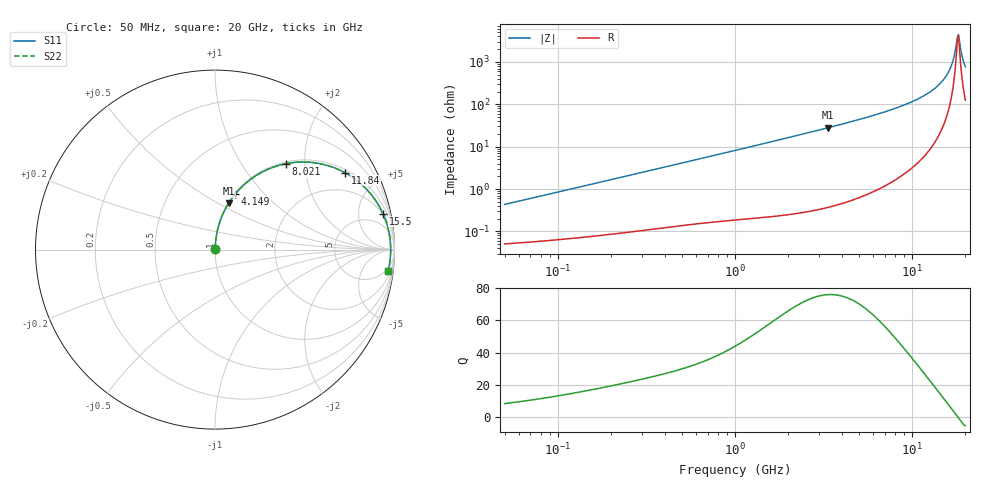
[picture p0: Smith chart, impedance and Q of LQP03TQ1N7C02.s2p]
!Murata Part Number: LQP03TQ1N7C02
!These Parameters are Measured in Series Mode Connection
!  o--[Z]--o
!Port1  Port2
!  o-------o
!Freq. Start=50[MHz] Stop=20[GHz], 401[Steps]
# Hz S RI R 50
!Freq.(Hz) S11(Real) S11(Imag) S21(Real) S21(Imag) S12(Real) S12(Imag) S22(Real) S22(Imag)
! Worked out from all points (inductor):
!   401 points, 50 MHz to 20 GHz, reference 50 ohm
!   read as one part in series: L = 1.36 nH near 51.52 MHz
!   highest Q = 75.9 at 3.364 GHz (marker M1), where L = 1.33 nH
!   self-resonance near 18.01 GHz
!   S11 on the Smith chart (normalised r, x): 50 MHz: 1.00, +0.01; 4.149 GHz: 1.01, +0.70; 8.021 GHz: 1.03, +1.60; 11.84 GHz: 1.12, +3.30; 15.5 GHz: 1.90, +9.01; 20 GHz: 4, -15
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5e7  0.000523 0.00429  0.9995 -0.00429  0.9995 -0.00429  0.000523 0.00429
1.364002e8  0.000849 0.0114  0.9992 -0.0114  0.9992 -0.0114  0.000849 0.0114
3.721004e8  0.0021 0.0305  0.9979 -0.0305  0.9979 -0.0305  0.0021 0.0305
1e9  0.00837 0.0804  0.9916 -0.0804  0.9916 -0.0804  0.00837 0.0804
2.728004e9  0.0507 0.2128  0.9493 -0.2128  0.9493 -0.2128  0.0507 0.2128
3.364474e9  0.0759 0.2583  0.9241 -0.2583  0.9241 -0.2583  0.0759 0.2583
4.149438e9  0.1137 0.3109  0.8863 -0.3109  0.8863 -0.3109  0.1137 0.3109
5.683258e9  0.208 0.3984  0.792 -0.3984  0.792 -0.3984  0.208 0.3984
7.442007e9  0.3438 0.4657  0.6562 -0.4657  0.6562 -0.4657  0.3438 0.4657
8.020766e9  0.3931 0.4784  0.6069 -0.4784  0.6069 -0.4784  0.3931 0.4784
9.892087e9  0.5592 0.4832  0.4408 -0.4832  0.4408 -0.4832  0.5592 0.4832
1.183995e10  0.7242 0.4284  0.2758 -0.4284  0.2758 -0.4284  0.7242 0.4284
1.375312e10  0.8554 0.3241  0.1446 -0.3241  0.1446 -0.3241  0.8554 0.3241
1.550395e10  0.9353 0.2011  0.0647 -0.2011  0.0647 -0.2011  0.9353 0.2011
1.670968e10  0.9661 0.1103  0.0339 -0.1103  0.0339 -0.1103  0.9661 0.1103
1.721783e10  0.9734 0.0721  0.0266 -0.0721  0.0266 -0.0721  0.9734 0.0721
1.774144e10  0.9777 0.0333  0.0223 -0.0333  0.0223 -0.0333  0.9777 0.0333
1.800918e10  0.9786 0.0137  0.0214 -0.0137  0.0214 -0.0137  0.9786 0.0137
1.828096e10  0.9788 -0.00589  0.0212 0.00589  0.0212 0.00589  0.9788 -0.00589
1.855685e10  0.9782 -0.0255  0.0218 0.0255  0.0218 0.0255  0.9782 -0.0255
1.940974e10  0.9717 -0.0837  0.0283 0.0837  0.0283 0.0837  0.9717 -0.0837
2e10  0.9636 -0.1217  0.0364 0.1217  0.0364 0.1217  0.9636 -0.1217
